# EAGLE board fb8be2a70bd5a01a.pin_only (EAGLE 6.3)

Size 62.48 x 81.28 mm. Coordinates in mm from the lower left corner, seen from the top.
Outline: 0,2.54 arc90 2.54,0 59.94,0 arc90 62.48,2.54 arc90 59.94,5.08 56.64,5.08 56.64,76.2 59.94,76.2 arc90 62.48,78.74 arc90 59.94,81.28 2.54,81.28 arc90 0,78.74 arc90 2.54,76.2 5.84,76.2 5.84,5.08 2.54,5.08 arc90 0,2.54
Outline: 16.26,24.89 16.26,19.56 46.23,19.56 46.23,24.89 16.26,24.89
Copper layers (1*16): Top 0.035mm / dielectric 1.5mm / Bottom 0.035mm
Design rules "adafruit": minimum track width 8mil, minimum drill 15.5mil, track to track 8mil, track to pad 8mil, pad to pad 8mil, via to via 8mil, smd to smd 8mil, copper to edge 10mil, drill to drill 8mil, minimum pad ring 10mil, minimum via ring 8mil, stop-mask expansion 4mil, vias tented up to drill 20mil, thermal gap 10mil

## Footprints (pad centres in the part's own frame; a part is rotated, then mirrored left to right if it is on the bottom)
0805-NO = smd 1.3 x 1.5: 1 -0.95,0; 2 0.95,0
SOT23-5L = smd 0.55 x 1.2: 1 -0.95,-1.3; 2 0,-1.3; 3 0.95,-1.3; 4 0.95,1.3; 5 -0.95,1.3
SO20W = smd 0.66 x 2.032: 1 -5.715,-5.029; 2 -4.445,-5.029; 3 -3.175,-5.029; 4 -1.905,-5.029; 5 -0.635,-5.029; 6 0.635,-5.029; 7 1.905,-5.029; 8 3.175,-5.029; 9 4.445,-5.029; 10 5.715,-5.029; 11 5.715,5.029; 12 4.445,5.029; 13 3.175,5.029; 14 1.905,5.029; 15 0.635,5.029; 16 -0.635,5.029; 17 -1.905,5.029; 18 -3.175,5.029; 19 -4.445,5.029; 20 -5.715,5.029
SOT23 = smd 1 x 1.4: 1 -0.95,-1.1; 2 0.95,-1.1; 3 0,1.1
1X20_ROUND = drill 1 pad 1.676 square: 1 -24.13,0 | drill 1 pad 1.676: 2 -21.59,0; 3 -19.05,0; 4 -16.51,0; 5 -13.97,0; 6 -11.43,0; 7 -8.89,0; 8 -6.35,0; 9 -3.81,0; 10 -1.27,0; 11 1.27,0; 12 3.81,0; 13 6.35,0; 14 8.89,0; 15 11.43,0; 16 13.97,0; 17 16.51,0; 18 19.05,0; 19 21.59,0; 20 24.13,0
SOT23-BEC = smd 1 x 1.4: B -0.95,-1.1; C 0,1.1; E 0.95,-1.1
R0805 = smd 1.3 x 1.5: 1 -0.95,0; 2 0.95,0
SOLDERJUMPER_ARROW_NOPASTE = smd 0.762 x 1.524: 1 -1.016,0; 2 1.016,0
MOUNTINGHOLE_3.0_PLATEDTHIN = drill 3 pad 3.6: P$1 0,0
FIDUCIAL_1MM = smd 1 x 1: 1 0,0
TFT_2.83IN_240X320_50PIN = smd 0.275 x 1.2 bottom: 1 12.25,-10.39; 2 11.75,-10.39; 3 11.25,-10.39; 4 10.75,-10.39; 5 10.25,-10.39; 6 9.75,-10.39; 7 9.25,-10.39; 8 8.75,-10.39; 9 8.25,-10.39; 10 7.75,-10.39; 11 7.25,-10.39; 12 6.75,-10.39; 13 6.25,-10.39; 14 5.75,-10.39; 15 5.25,-10.39; 16 4.75,-10.39; 17 4.25,-10.39; 18 3.75,-10.39; 19 3.25,-10.39; 20 2.75,-10.39; 21 2.25,-10.39; 22 1.75,-10.39; 23 1.25,-10.39; 24 0.75,-10.39; 25 0.25,-10.39; 26 -0.25,-10.39; 27 -0.75,-10.39; 28 -1.25,-10.39; 29 -1.75,-10.39; 30 -2.25,-10.39; 31 -2.75,-10.39; 32 -3.25,-10.39; 33 -3.75,-10.39; 34 -4.25,-10.39; 35 -4.75,-10.39; 36 -5.25,-10.39; 37 -5.75,-10.39; 38 -6.25,-10.39; 39 -6.75,-10.39; 40 -7.25,-10.39; 41 -7.75,-10.39; 42 -8.25,-10.39; 43 -8.75,-10.39; 44 -9.25,-10.39; 45 -9.75,-10.39; 46 -10.25,-10.39; 47 -10.75,-10.39; 48 -11.25,-10.39; 49 -11.75,-10.39; 50 -12.25,-10.39 | smd 2.4 x 2.4 bottom: PAD1 14.35,-13.09; PAD2 -14.35,-13.09
MICROSD = smd 0.7 x 1.5: 1 9,-10.64; 2 7.9,-10.24; 3 6.8,-10.64; 4 5.7,-11.04; 5 4.6,-10.64; 6 3.5,-11.04; 7 2.4,-10.64; 8 1.3,-10.64 | smd 1.8 x 1.4: CD1 2,-0.44; CD2 8,-0.44 | smd 1.4 x 1.9: MT1 0.4,-13.54; MT2 13.6,-14.44

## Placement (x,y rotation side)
C1  0.1uF  [0805-NO]  12.45,49.28 180 top
C2  10uF  [0805-NO]  53.85,9.65 0 top
C3  10uF  [0805-NO]  50.8,45.47 0 top
C4  0.1uF  [0805-NO]  25.91,38.61 270 top
C5  10uF  [0805-NO]  52.58,35.81 180 top
IC1  MIC5225-3.3  [SOT23-5L]  50.8,40.89 0 top
IC2  74LVC245  [SO20W]  31.5,59.18 180 top
IC3  74LVC245  [SO20W]  46.48,58.93 180 top
IC4  APX803-SAG  [SOT23]  36.83,49.78 0 top
JP1  [1X20_ROUND]  31.24,78.74 180 top
JP2  [1X20_ROUND]  31.24,2.54 180 top
Q1  MMBT2222  [SOT23-BEC]  14.48,38.35 180 top
R1  10  [0805-NO]  17.53,38.61 270 top
R2  10  [0805-NO]  19.56,38.61 270 top
R3  10  [0805-NO]  21.59,38.61 270 top
R4  10  [0805-NO]  23.62,38.61 270 top
R5  1K  [0805-NO]  14.48,42.16 0 top
R6  10K  [R0805]  39.62,50.55 90 top
R7  1K  [0805-NO]  39.75,68.2 0 top
R8  10K  [0805-NO]  8.76,13.21 90 top
R9  10K  [0805-NO]  11.18,12.57 90 top
R10  10K  [0805-NO]  16.38,12.57 270 top
R11  10K  [0805-NO]  13.72,12.57 270 top
R12  10K  [0805-NO]  38.99,64.14 270 top
SJ1  [SOLDERJUMPER_ARROW_NOPASTE]  8.89,29.72 180 top
SJ2  [SOLDERJUMPER_ARROW_NOPASTE]  8.89,33.53 180 top
SJ3  [SOLDERJUMPER_ARROW_NOPASTE]  8.89,37.47 0 top
SJ4  [SOLDERJUMPER_ARROW_NOPASTE]  8.89,41.53 0 top
U$7  MOUNTINGHOLE3.0THIN  [MOUNTINGHOLE_3.0_PLATEDTHIN]  2.67,2.54 0 top
U$9  FIDUCIAL  [FIDUCIAL_1MM]  54.86,25.15 0 top
U$10  DISP_LCD_1.28IN_240X320_50PIN  [TFT_2.83IN_240X320_50PIN]  31.24,43.18 0 bottom
U$11  FIDUCIAL  [FIDUCIAL_1MM]  8.89,69.09 0 top
U$15  MOUNTINGHOLE3.0THIN  [MOUNTINGHOLE_3.0_PLATEDTHIN]  59.82,2.54 0 top
U$16  MOUNTINGHOLE3.0THIN  [MOUNTINGHOLE_3.0_PLATEDTHIN]  2.67,78.74 0 top
U$17  MOUNTINGHOLE3.0THIN  [MOUNTINGHOLE_3.0_PLATEDTHIN]  59.82,78.74 0 top
U$19  [ADAFRUIT_TEXT_30MM]  18.8,39.62 0 top
U$23  FIDUCIAL  [FIDUCIAL_1MM]  15.24,32.77 0 top
X1  [MICROSD]  22.86,66.29 270 top

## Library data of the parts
C1-C5 JP1 JP2 R1-R5 R7-R12 U$10 U$19 X1 = microbuilder
IC1 IC4 U$9 U$11 U$23 = adafruit
IC2 IC3 = 74xx-eu
Q1 = transistor-neu-to92
R6 = rcl
SJ1-SJ4 U$7 U$15-U$17 = microbuilder; BOM: EXCLUDE

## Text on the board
tPlace: D7 | D6 | D5 | D4 | D3 | D2 | D1 | D0 | Y- | X- | Y+ | X+ | Backlite | RST | RD | WR | C/D | CS | 3-5V | GND | LCD Data I/O | Touchscreen | LCD control | PWR | Inputs | Bi-directional | 8-bit 8080-type parallel | IM3 | IM2 | IM1 | ILI9341 | IM0 | Close IM1/IM2/IM3 / for SPI | 2.8" TFT LCD Breakout Board+ | 4-wire Resistive Touchscreen | Power with 3.3V-5V | v2.3 | Logic at 3.3V-5V | SPI Interface | Card Detect | Card CS | IM0 | IM1 | IM2 | IM3 | X- | Y- | X+ | Y+ | Lite | RST | D/C | CS | MOSI | MISO | CLK | 3.3V out | 3-5V | GND
bPlace: Lite | RD | C/D | Vin | D7 | D6 | D5 | D4 | D3 | D2 | D1 | D0 | Y- | X- | Y+ | X+ | RST | WR | CS | GND | CD | IM0 | IM2 | X- | X+ | Lite | D/C | MOSI | CLK | Vin | CCS | IM1 | IM3 | Y- | Y+ | RST | CS | MISO | 3Vo | GND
